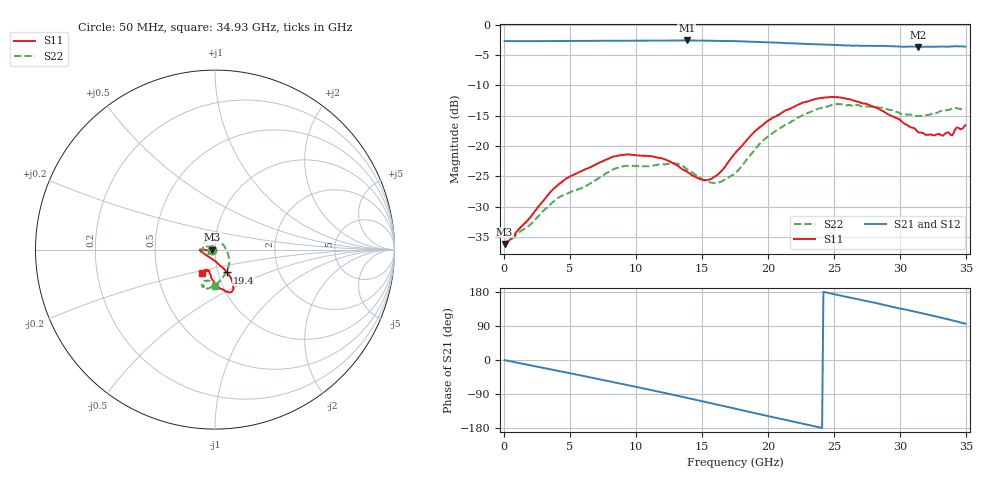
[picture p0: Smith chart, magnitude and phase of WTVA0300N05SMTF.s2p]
! 50 ohm 2-Port S-parameters measured by Modelithics Inc support@modelithics.com  Tampa, FL USA 813-866-6335 (February 2024)
! Smiths Interconnect,  3dB P/N: WTVA0300N05SMTF, Temperature: 50 C
! Board: 10 mil Rogers 4350B, Mounting Pad Dimensions: Length: 15 mils, Width: 25 mils, Gap: 40 mils.
# Hz S RI R 50
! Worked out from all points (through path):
!   352 points, 50 MHz to 34.93 GHz, reference 50 ohm
!   highest |S21| = -2.59 dB at 13.83 GHz (marker M1); lowest = -3.7 dB at 31.34 GHz (marker M2)
!   group delay of S21, straight-line fit = 21.1 ps
!   lowest |S11| = -36.2 dB at 50 MHz (marker M3), VSWR 1.03, Z = 48.5 + j0.0337 ohm
!   |S11| at or under -10 dB: start of sweep to end of sweep
!   |S22| runs from -36.5 to -13.1 dB; largest |S21 - S12| = 0.0081
!   S11 on the Smith chart (normalised r, x): 50 MHz: 0.97, +0.00; 19.4 GHz: 1.10, -0.29; 34.93 GHz: 0.84, -0.22
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5e7  -0.0155 0.000347  0.7327 -0.00404  0.732 -0.004  -0.0148 -0.00108
3.6825e9  -0.0434 -0.00384  0.6625 -0.3165  0.6617 -0.3169  -0.0279 -0.02
5.8715e9  -0.062 -0.000321  0.5549 -0.4844  0.5545 -0.4841  -0.0373 -0.0248
8.6575e9  -0.0833 0.000709  0.3563 -0.6462  0.3552 -0.6462  -0.0641 -0.0172
1.1742e10  -0.0791 -0.0107  0.0798 -0.7355  0.0783 -0.735  -0.0643 0.0286
1.30355e10  -0.0674 -0.0182  -0.0457 -0.7394  -0.047 -0.7389  -0.0516 0.0497
1.38315e10  -0.0551 -0.0273  -0.1257 -0.7315  -0.1259 -0.731  -0.0325 0.0557
1.48265e10  -0.0367 -0.0384  -0.2223 -0.7067  -0.2234 -0.7057  -0.00508 0.0547
1.5722e10  -0.0182 -0.0504  -0.3061 -0.6713  -0.3064 -0.6704  0.0215 0.0448
1.66175e10  0.00206 -0.0647  -0.3833 -0.627  -0.3841 -0.626  0.0433 0.0291
1.7513e10  0.0223 -0.0847  -0.4561 -0.5735  -0.4562 -0.5727  0.0594 0.00441
1.94035e10  0.0672 -0.1271  -0.5794 -0.4298  -0.5785 -0.43  0.08 -0.0689
2.1294e10  0.0945 -0.1717  -0.6552 -0.2615  -0.6548 -0.2612  0.0557 -0.1386
2.33835e10  0.1028 -0.2176  -0.6889 -0.0736  -0.6884 -0.0738  0.00144 -0.1949
2.5075e10  0.085 -0.2382  -0.6769 0.0817  -0.6762 0.0838  -0.0412 -0.217
2.61695e10  0.064 -0.2341  -0.6504 0.1757  -0.6495 0.1773  -0.063 -0.2085
2.91545e10  -0.00513 -0.1802  -0.5277 0.408  -0.5235 0.4123  -0.0681 -0.1867
3.13435e10  -0.0298 -0.1267  -0.3817 0.5345  -0.3784 0.5361  -0.0341 -0.1732
3.39305e10  -0.0504 -0.1114  -0.169 0.6402  -0.1644 0.6408  -0.00166 -0.2027
3.4229e10  -0.0608 -0.1261  -0.1396 0.6501  -0.1345 0.6505  -0.00544 -0.2047
3.4627e10  -0.0605 -0.1235  -0.0946 0.6561  -0.0948 0.6553  -0.00389 -0.2012
3.49255e10  -0.0706 -0.1305  -0.0661 0.6571  -0.0659 0.6563  0.00215 -0.2039
